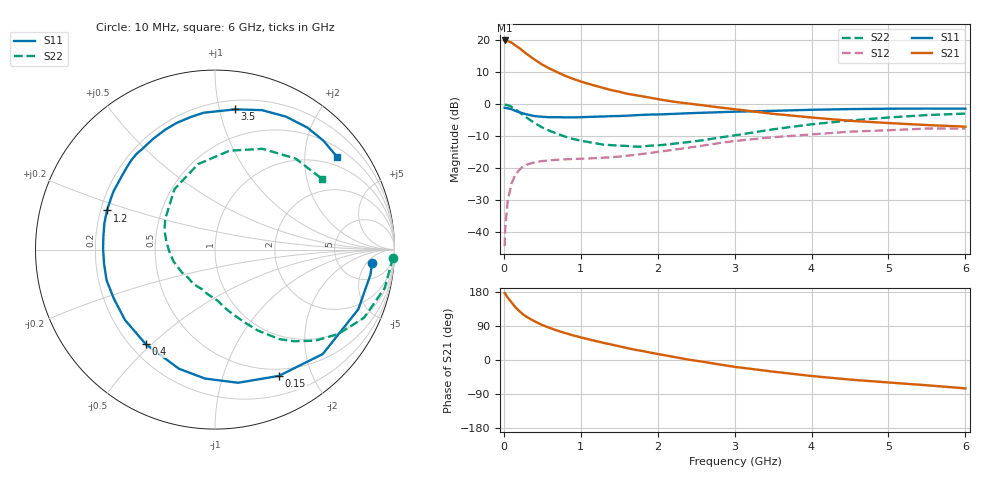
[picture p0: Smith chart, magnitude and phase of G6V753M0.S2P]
! SIEMENS Small Signal Semiconductors
! BFG193
! Si NPN RF Bipolar Junction Transistor in SOT223
! VCE = 0.75 V  IC = 3 mA
! Common Emitter S-Parameters:  August  1996
# GHz  S  MA  R  50
!  f  S11  S21  S12  S22
! GHz  MAG  ANG  MAG  ANG  MAG  ANG  MAG  ANG
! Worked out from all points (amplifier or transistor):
!   36 points, 10 MHz to 6 GHz, reference 50 ohm
!   highest |S21| = 20.0 dB at 10 MHz (marker M1)
!   |S21| within 3 dB of that: start of sweep to 233 MHz
!   unconditionally stable (mu >= 1): 1.225 GHz to 3.536 GHz; 5.971778 GHz to end of sweep
!   at 250 MHz: K = 0.25, MSG = 18.1 dB, |S12| = -19.5 dB
!   at 1.4 GHz: K = 1.09, MAG = 8.7 dB, |S12| = -16.6 dB
!   at 6 GHz: K = 1.00, MAG = 0.1 dB, |S12| = -7.6 dB
!   S11 on the Smith chart (normalised r, x): 10 MHz: 11, -7; 150 MHz: 0.42, -1.55; 400 MHz: 0.26, -0.48; 1.2 GHz: 0.23, +0.17; 3.5 GHz: 0.27, +1.12; 6 GHz: 0.73, +2.79
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0.01  0.8799 -4.8  9.98 176.9  0.006 89.9  0.9914 -2.6
0.02  0.8769 -9.3  9.966 174.8  0.0121 84.7  0.984 -5.1
0.05  0.8649 -22.6  9.796 164.6  0.0305 77.4  0.9691 -12.8
0.1  0.836 -44.1  9.233 152.1  0.0578 66.7  0.9136 -24.5
0.15  0.7886 -63.1  8.338 139.1  0.0786 56.2  0.832 -34.5
0.2  0.7532 -80.1  7.602 129.5  0.0938 49.4  0.755 -42.2
0.25  0.7205 -94.5  6.804 120.5  0.1057 42.6  0.6745 -49.2
0.3  0.6933 -106.9  6.101 113.4  0.1137 38.1  0.6141 -54.3
0.4  0.653 -126.2  5.004 102.1  0.1236 31.0  0.5078 -62.3
0.5  0.6364 -142.0  4.174 92.2  0.129 26.1  0.4326 -68.3
0.6  0.6263 -154.2  3.598 84.4  0.1328 23.2  0.3816 -73.5
0.7  0.6278 -164.3  3.154 77.3  0.1353 21.0  0.3434 -78.4
0.9  0.6239 179.1  2.503 65.1  0.1391 18.8  0.2862 -86.8
1.1  0.6338 166.3  2.089 54.7  0.1416 18.1  0.256 -97.4
1.2  0.64 160.1  1.933 49.8  0.1436 18.1  0.2444 -102.6
1.6  0.6624 141.2  1.464 31.5  0.1567 19.0  0.2223 -126.0
2.2  0.7068 119.2  1.1 8.5  0.1933 18.2  0.2403 -164.1
2.8  0.7509 100.4  0.893 -11.7  0.247 11.8  0.301 159.2
3.5  0.7892 81.9  0.709 -30.7  0.305 -2.4  0.4053 123.9
4.5  0.8399 61.9  0.551 -51.7  0.3725 -22.1  0.5566 81.7
5.5  0.8563 45.1  0.473 -66.7  0.4164 -46.1  0.6777 48.4
6  0.8539 37.3  0.446 -74.9  0.4165 -59.6  0.7139 33.6
